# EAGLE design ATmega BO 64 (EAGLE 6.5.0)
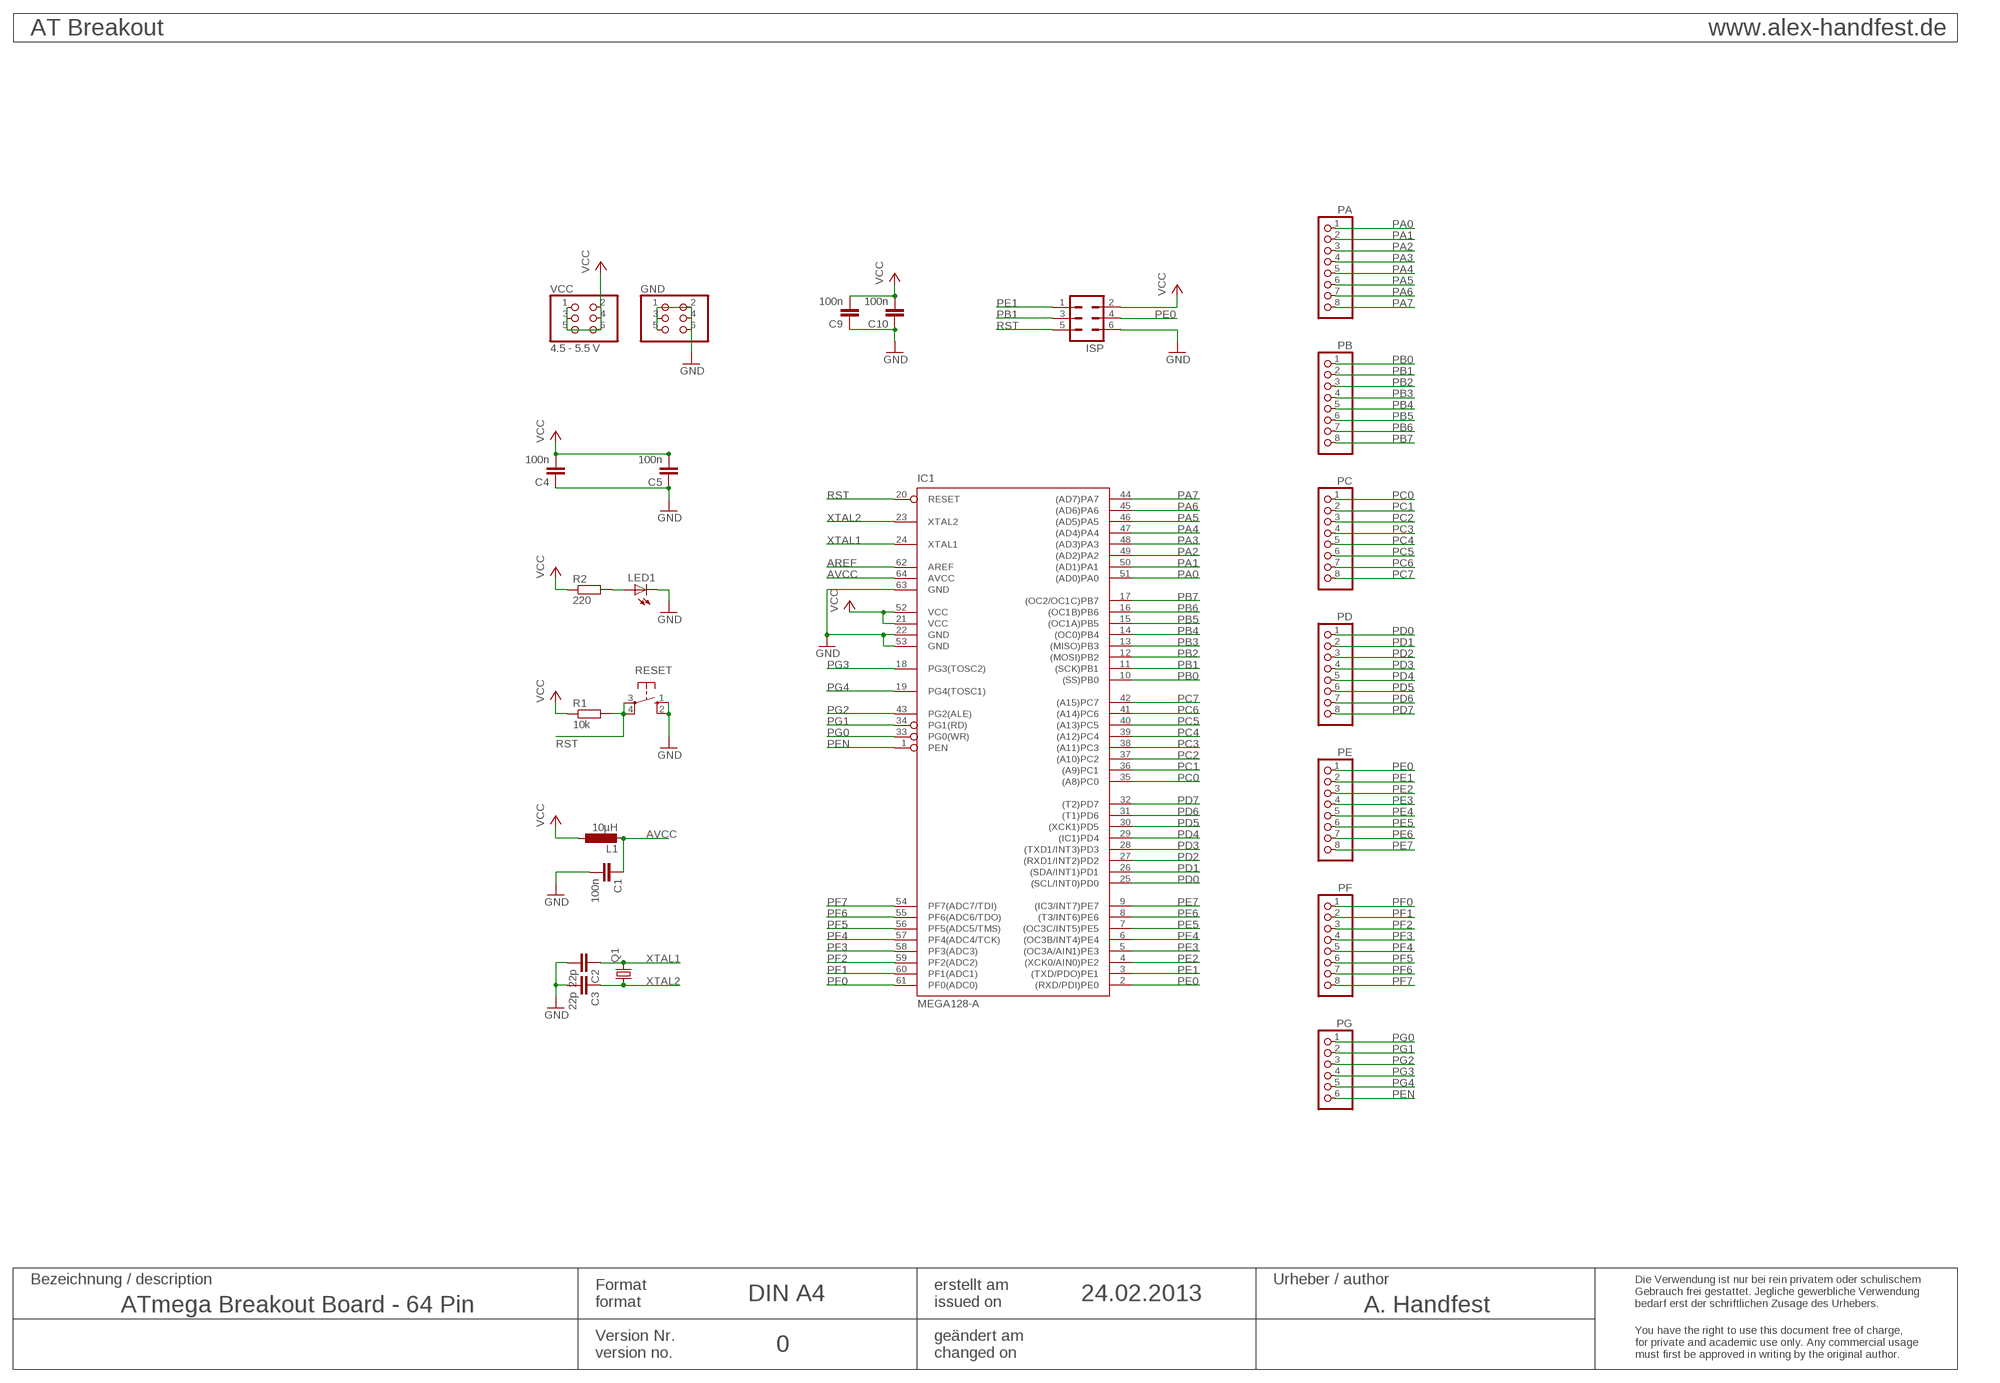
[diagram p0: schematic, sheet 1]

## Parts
C1  100n  C-EUC0805  [C0805]
C2  22p  C-EUC0805  [C0805]
C3  22p  C-EUC0805  [C0805]
C4  100n  C-EUC0805  [C0805]
C5  100n  C-EUC0805  [C0805]
C9  100n  C-EUC0805  [C0805]
C10  100n  C-EUC0805  [C0805]
GND  PINHD-2X3  [2X03]
IC1  MEGA128-A  [TQFP64]
ISP  ML6  [ML6]
L1  10µH  L-EUL2012C  [L2012C]
LED1  LEDCHIP-LED0805  [CHIP-LED0805]
PA  PINHD-1X8  [1X08]
PB  PINHD-1X8  [1X08]
PC  PINHD-1X8  [1X08]
PD  PINHD-1X8  [1X08]
PE  PINHD-1X8  [1X08]
PF  PINHD-1X8  [1X08]
PG  PINHD-1X6  [1X06]
Q1  CRYSTALCTS406  [CTS406]
R1  10k  R-EU_R0805  [R0805]
R2  220  R-EU_R0805  [R0805]
RESET  10-XX  [B3F-10XX]
VCC  4.5 - 5.5 V  PINHD-2X3  [2X03]

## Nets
AREF: IC1.62(AREF)
AVCC: C1.1 IC1.64(AVCC) L1.2
GND: C1.2 C2.2 C3.2 C4.1 C5.1 C9.1 C10.1 GND.1 GND.2 GND.3 GND.4 GND.5 GND.6 IC1.22(GND) IC1.53(GND) IC1.63(GND) ISP.6 LED1.C RESET.1(S) RESET.2(S1)
N$6: LED1.A R2.2
PA0: IC1.51((AD0)PA0) PA.1
PA1: IC1.50((AD1)PA1) PA.2
PA2: IC1.49((AD2)PA2) PA.3
PA3: IC1.48((AD3)PA3) PA.4
PA4: IC1.47((AD4)PA4) PA.5
PA5: IC1.46((AD5)PA5) PA.6
PA6: IC1.45((AD6)PA6) PA.7
PA7: IC1.44((AD7)PA7) PA.8
PB0: IC1.10((SS)PB0) PB.1
PB1: IC1.11((SCK)PB1) ISP.3 PB.2
PB2: IC1.12((MOSI)PB2) PB.3
PB3: IC1.13((MISO)PB3) PB.4
PB4: IC1.14((OC0)PB4) PB.5
PB5: IC1.15((OC1A)PB5) PB.6
PB6: IC1.16((OC1B)PB6) PB.7
PB7: IC1.17((OC2/OC1C)PB7) PB.8
PC0: IC1.35((A8)PC0) PC.1
PC1: IC1.36((A9)PC1) PC.2
PC2: IC1.37((A10)PC2) PC.3
PC3: IC1.38((A11)PC3) PC.4
PC4: IC1.39((A12)PC4) PC.5
PC5: IC1.40((A13)PC5) PC.6
PC6: IC1.41((A14)PC6) PC.7
PC7: IC1.42((A15)PC7) PC.8
PD0: IC1.25((SCL/INT0)PD0) PD.1
PD1: IC1.26((SDA/INT1)PD1) PD.2
PD2: IC1.27((RXD1/INT2)PD2) PD.3
PD3: IC1.28((TXD1/INT3)PD3) PD.4
PD4: IC1.29((IC1)PD4) PD.5
PD5: IC1.30((XCK1)PD5) PD.6
PD6: IC1.31((T1)PD6) PD.7
PD7: IC1.32((T2)PD7) PD.8
PE0: IC1.2((RXD/PDI)PE0) ISP.4 PE.1
PE1: IC1.3((TXD/PDO)PE1) ISP.1 PE.2
PE2: IC1.4((XCK0/AIN0)PE2) PE.3
PE3: IC1.5((OC3A/AIN1)PE3) PE.4
PE4: IC1.6((OC3B/INT4)PE4) PE.5
PE5: IC1.7((OC3C/INT5)PE5) PE.6
PE6: IC1.8((T3/INT6)PE6) PE.7
PE7: IC1.9((IC3/INT7)PE7) PE.8
PEN: IC1.1(PEN) PG.6
PF0: IC1.61(PF0(ADC0)) PF.1
PF1: IC1.60(PF1(ADC1)) PF.2
PF2: IC1.59(PF2(ADC2)) PF.3
PF3: IC1.58(PF3(ADC3)) PF.4
PF4: IC1.57(PF4(ADC4/TCK)) PF.5
PF5: IC1.56(PF5(ADC5/TMS)) PF.6
PF6: IC1.55(PF6(ADC6/TDO)) PF.7
PF7: IC1.54(PF7(ADC7/TDI)) PF.8
PG0: IC1.33(PG0(WR)) PG.1
PG1: IC1.34(PG1(RD)) PG.2
PG2: IC1.43(PG2(ALE)) PG.3
PG3: IC1.18(PG3(TOSC2)) PG.4
PG4: IC1.19(PG4(TOSC1)) PG.5
RST: IC1.20(RESET) ISP.5 R1.2 RESET.3(P) RESET.4(P1)
VCC: C4.2 C5.2 C9.2 C10.2 IC1.21(VCC) IC1.52(VCC) ISP.2 L1.1 R1.1 R2.1 VCC.1 VCC.2 VCC.3 VCC.4 VCC.5 VCC.6
XTAL1: C2.1 IC1.24(XTAL1) Q1.3
XTAL2: C3.1 IC1.23(XTAL2) Q1.1

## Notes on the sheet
- AT Breakout | www.alex-handfest.de
- Bezeichnung / description | Urheber / author
- Format | erstellt am
- DIN A4 | 24.02.2013
- format | issued on
- Die Verwendung ist nur bei rein privatem oder schulischem
  Gebrauch frei gestattet. Jegliche gewerbliche Verwendung 
  bedarf erst der schriftlichen Zusage des Urhebers.
- ATmega Breakout Board - 64 Pin | A. Handfest
- Version Nr. | geändert am
- 0
- version no. | changed on
- You have the right to use this document free of charge,
  for private and academic use only. Any commercial usage
  must first be approved in writing by the original author.

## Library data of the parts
C1-C5 C9 C10 = rcl:C-EU: CAPACITOR, European symbol
GND VCC = pinhead:PINHD-2X3: PIN HEADER
IC1 = atmel:MEGA128: MICROCONTROLLER 128 Kbytes FLASH 4 Kbytes SRAM 4 Kbytes EEPROM DUAL USART 8-channel 10 bit ADC Source: avr.lbr
ISP = con-harting-ml:ML6: HARTING
L1 = rcl:L-EU: INDUCTOR, European symbol
LED1 = led:LED: LED
PA PB PC PD PE PF = pinhead:PINHD-1X8: PIN HEADER
PG = pinhead:PINHD-1X6: PIN HEADER
Q1 = crystal:CRYSTAL: CRYSTAL; OC_FARNELL: unknown; OC_NEWARK: unknown
R1 R2 = rcl:R-EU_: RESISTOR, European symbol
RESET = switch-omron:10-XX: OMRON SWITCH

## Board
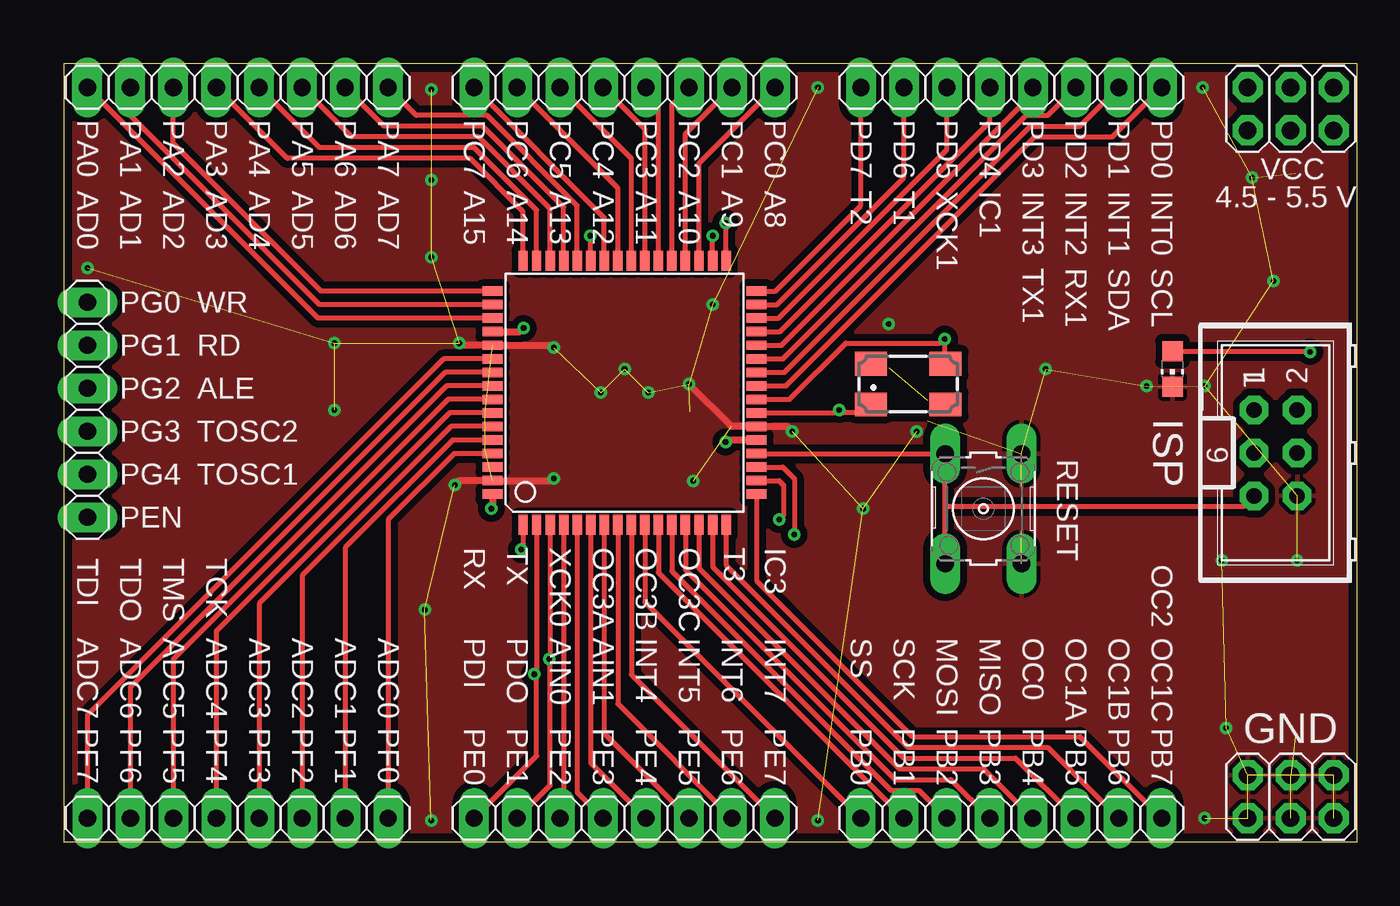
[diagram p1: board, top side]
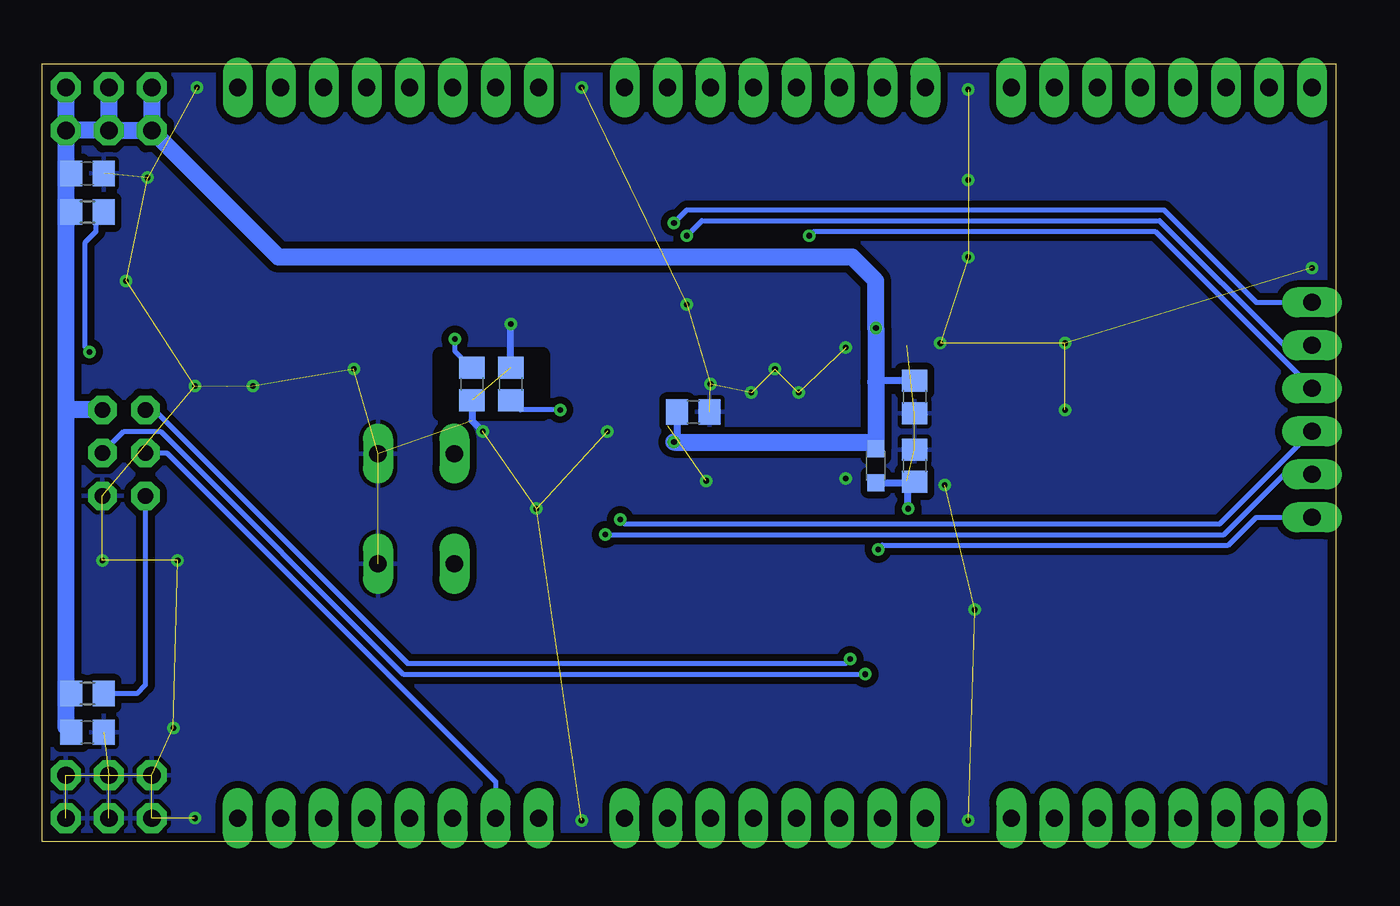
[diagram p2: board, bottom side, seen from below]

Size 76.45 x 45.97 mm. Coordinates in mm from the lower left corner, seen from the top.
Outline: 0,0 76.45,0 76.45,45.97 0,45.97 0,0
Copper layers (1*16): Top 0.035mm / dielectric 1.5mm / Bottom 0.035mm
Design rules "default *": minimum track width 10mil, minimum drill 24mil, track to track 8mil, track to pad 8mil, pad to pad 8mil, via to via 8mil, smd to smd 8mil, copper to edge 20mil, drill to drill 8mil, minimum pad ring 15mil, minimum via ring 8mil, stop-mask expansion 4mil, vias tented up to drill 20mil, thermal gap 10mil
tRestrict: area 46.9,25.3 to 53,28.8
bRestrict: area 46.9,25.3 to 53,28.8

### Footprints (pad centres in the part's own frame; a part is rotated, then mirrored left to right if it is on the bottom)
C0805 = smd 1.3 x 1.5: 1 -0.95,0; 2 0.95,0
2X03 = drill 1.016 octagon: 1 -2.54,-1.27; 2 -2.54,1.27; 3 0,-1.27; 4 0,1.27; 5 2.54,-1.27; 6 2.54,1.27
TQFP64 = smd 1.194 x 0.559: 1 -7.8,6; 2 -7.8,5.2; 3 -7.8,4.4; 4 -7.8,3.6; 5 -7.8,2.8; 6 -7.8,2; 7 -7.8,1.2; 8 -7.8,0.4; 9 -7.8,-0.4; 10 -7.8,-1.2; 11 -7.8,-2; 12 -7.8,-2.8; 13 -7.8,-3.6; 14 -7.8,-4.4; 15 -7.8,-5.2; 16 -7.8,-6; 33 7.8,-6; 34 7.8,-5.2; 35 7.8,-4.4; 36 7.8,-3.6; 37 7.8,-2.8; 38 7.8,-2; 39 7.8,-1.2; 40 7.8,-0.4; 41 7.8,0.4; 42 7.8,1.2; 43 7.8,2; 44 7.8,2.8; 45 7.8,3.6; 46 7.8,4.4; 47 7.8,5.2; 48 7.8,6 | smd 0.559 x 1.194: 17 -6,-7.8; 18 -5.2,-7.8; 19 -4.4,-7.8; 20 -3.6,-7.8; 21 -2.8,-7.8; 22 -2,-7.8; 23 -1.2,-7.8; 24 -0.4,-7.8; 25 0.4,-7.8; 26 1.2,-7.8; 27 2,-7.8; 28 2.8,-7.8; 29 3.6,-7.8; 30 4.4,-7.8; 31 5.2,-7.8; 32 6,-7.8; 49 6,7.8; 50 5.2,7.8; 51 4.4,7.8; 52 3.6,7.8; 53 2.8,7.8; 54 2,7.8; 55 1.2,7.8; 56 0.4,7.8; 57 -0.4,7.8; 58 -1.2,7.8; 59 -2,7.8; 60 -2.8,7.8; 61 -3.6,7.8; 62 -4.4,7.8; 63 -5.2,7.8; 64 -6,7.8
ML6 = drill 0.914 octagon: 1 -2.54,-1.27; 2 -2.54,1.27; 3 0,-1.27; 4 0,1.27; 5 2.54,-1.27; 6 2.54,1.27
L2012C = smd 1 x 1: 1 -1,0; 2 1,0
CHIP-LED0805 = smd 1.2 x 1.2: A 0,-1.05; C 0,1.05
1X08 = drill 1.016 long: 1 -8.89,0; 2 -6.35,0; 3 -3.81,0; 4 -1.27,0; 5 1.27,0; 6 3.81,0; 7 6.35,0; 8 8.89,0
1X06 = drill 1.016 long: 1 -6.35,0; 2 -3.81,0; 3 -1.27,0; 4 1.27,0; 5 3.81,0; 6 6.35,0
CTS406 = smd 1.9 x 1.4: 1 -2.2,-1.2; 2 2.2,-1.2; 3 2.2,1.2; 4 -2.2,1.2
R0805 = smd 1.3 x 1.5: 1 -0.95,0; 2 0.95,0
B3F-10XX = drill 1.016 long: 1 -3.251,2.261; 2 3.251,2.261; 3 -3.251,-2.261; 4 3.251,-2.261

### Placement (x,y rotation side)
C1  24.89,22.23 90 bottom
C2  51.05,27.05 270 bottom
C3  48.77,27.05 90 bottom
C4  37.97,25.4 180 bottom
C5  24.89,26.29 90 bottom
C9  73.79,6.48 180 bottom
C10  73.79,39.5 180 bottom
GND  72.52,2.67 0 top
IC1  33.15,26.54 90 top
ISP  71.63,22.99 270 top
L1  27.18,22.23 270 bottom
LED1  65.53,27.94 180 top
PA  10.29,44.58 0 top
PB  56.01,1.4 0 top
PC  33.15,44.58 180 top
PD  56.01,44.58 180 top
PE  33.15,1.4 0 top
PF  10.29,1.4 180 top
PG  1.4,25.53 270 top
Q1  49.91,27.05 0 top
R1  73.79,8.76 0 bottom
R2  73.79,37.21 0 bottom
RESET  54.36,19.68 270 top
VCC  72.52,43.31 0 top

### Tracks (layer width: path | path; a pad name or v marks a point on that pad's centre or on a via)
AVCC  (via drill 0.33)
  Top 0.406: IC1.64 25.35,19.76 v25.27,19.68
  Bottom 0.406: L1.2 25.4,21.23 | 25.4,21.23 24.94,21.23 C1.1 | v25.27,19.68 25.27,21.1 25.4,21.23
GND  (via drill 0.33)  (45 unrouted)
  Top 0.406: v23.37,29.46 23.49,29.34 IC1.53 28.82,29.34 v28.96,29.21 | v23.11,21.08 23.38,21.34 IC1.63 28.84,21.34 v28.96,21.46 | v36.96,27.05 39.47,24.54 IC1.22 42.77,24.54 v43.05,24.26
  Bottom 0.406: C2.2 51.05,24.89 v50.42,24.26 | C3.2 v48.77,30.61
  other vias: 31.75,26.54 33.15,27.94 34.54,26.54 37.21,21.34 38.35,31.75 70.23,39.24 67.44,26.92 64.01,26.92 72.9,16.64 68.45,16.64 68.71,6.73 44.58,1.27 67.44,1.4 21.72,1.27 1.4,33.91 21.72,44.45 21.72,39.12 21.72,34.54 16,29.46 16,25.53 44.58,44.58 67.31,44.58 58.04,27.94 47.24,19.68 21.34,13.72 71.5,33.15
  pour Bottom (isolate 0.406): -0.25,46.23 76.71,46.23 76.71,-0.25 -0.25,-0.25
  pour Top (isolate 0.406): -0.25,46.23 76.71,46.23 76.71,-0.25 -0.25,-0.25
N$6  (via drill 0.33)
  Top 0.305: LED1.A 73.63,28.99 v73.66,28.96
  Bottom 0.305: v73.66,28.96 73.91,29.21 73.91,35.43 73.28,36.07 73.28,36.77 R2.2
PA0
  Top 0.305: IC1.51 15.03,30.94 PA.1
PA1
  Top 0.305: IC1.50 15.12,31.74 3.94,42.93 PA.2
PA2
  Top 0.305: IC1.49 15.21,32.54 6.48,41.27 PA.3
PA3
  Top 0.305: IC1.48 27.15,37.24 24,40.39 13.21,40.39 PA.4
PA4
  Top 0.305: IC1.47 27.95,37.33 24.26,41.02 15.11,41.02 PA.5
PA5
  Top 0.305: IC1.46 28.75,37.42 24.51,41.66 17.02,41.66 PA.6
PA6
  Top 0.305: IC1.45 29.55,37.51 24.77,42.29 18.92,42.29 PA.7
PA7
  Top 0.305: IC1.44 30.35,37.6 25.02,42.93 20.83,42.93 PA.8
PB0
  Top 0.305: IC1.10 34.35,14.17 PB.1
PB1
  Top 0.305: IC1.11 35.15,15.91 PB.2
  Bottom 0.305: ISP.3 69.09,22.99 49.66,3.56 PB.2
PB2
  Top 0.305: IC1.12 35.95,16 48.9,3.05 50.55,3.05 PB.3
PB3
  Top 0.305: IC1.13 36.75,16.09 49.15,3.68 52.45,3.68 PB.4
PB4
  Top 0.305: IC1.14 37.55,16.17 49.4,4.32 54.36,4.32 PB.5
PB5
  Top 0.305: IC1.15 38.35,16.26 49.66,4.95 56.26,4.95 PB.6
PB6
  Top 0.305: IC1.16 39.15,16.35 49.91,5.59 58.17,5.59 PB.7
PB7
  Top 0.305: IC1.17 40.95,15.44 50.16,6.22 60.07,6.22 PB.8
PC0
  Top 0.305: IC1.35 37.55,40.09 PC.1
PC1
  Top 0.305: IC1.36 36.75,41.83 PC.2
PC2
  Top 0.305: IC1.37 35.95,43.57 PC.3
PC3
  Top 0.305: IC1.38 35.15,43.85 PC.4
PC4
  Top 0.305: IC1.39 34.35,42.11 PC.5
PC5
  Top 0.305: IC1.40 33.55,40.37 PC.6
PC6
  Top 0.305: IC1.41 32.75,38.63 PC.7
PC7
  Top 0.305: IC1.42 31.95,36.89 PC.8
PD0
  Top 0.305: IC1.25 42.69,26.94 57.4,41.66 61.98,41.66 PD.1
PD1
  Top 0.305: IC1.26 42.6,27.74 57.15,42.29 60.07,42.29 PD.2
PD2
  Top 0.305: IC1.27 42.51,28.54 56.9,42.93 58.17,42.93 PD.3
PD3
  Top 0.305: IC1.28 42.42,29.34 57.28,44.2 PD.4
PD4
  Top 0.305: IC1.29 42.34,30.14 54.74,42.55 PD.5
PD5
  Top 0.305: IC1.30 42.25,30.94 52.2,40.89 PD.6
PD6
  Top 0.305: IC1.31 42.16,31.74 49.66,39.24 PD.7
PD7
  Top 0.305: IC1.32 42.07,32.54 47.12,37.59 PD.8
PE0  (via drill 0.33)
  Top 0.305: PE.1 27.95,5.09 27.95,9.77 v27.81,9.91 27.95,10.04 IC1.2
  Bottom 0.305: ISP.4 71.63,24.26 69.47,24.26 55.12,9.91 v27.81,9.91
PE1  (via drill 0.33)
  Top 0.305: PE.2 28.75,3.35 28.75,10.75 v28.7,10.79 28.75,10.84 IC1.3
  Bottom 0.305: ISP.1 69.85,25.53 54.86,10.54 28.96,10.54 v28.7,10.79
PE2
  Top 0.305: IC1.4 29.55,1.61 PE.3
PE3
  Top 0.305: IC1.5 30.35,2.93 PE.4
PE4
  Top 0.305: IC1.6 31.15,4.67 PE.5
PE5
  Top 0.305: IC1.7 31.95,6.41 PE.6
PE6
  Top 0.305: IC1.8 32.75,8.15 PE.7
PE7
  Top 0.305: IC1.9 33.55,9.89 PE.8
PEN  (via drill 0.33)
  Top 0.305: IC1.1 27.15,17.37 v27.05,17.27
  Bottom 0.305: v27.05,17.27 26.8,17.53 6.35,17.53 4.7,19.18 PG.6
PF0
  Top 0.305: IC1.61 23.07,22.94 19.18,19.05 PF.1
PF1
  Top 0.305: IC1.60 22.98,23.74 16.64,17.4 PF.2
PF2
  Top 0.305: IC1.59 22.89,24.54 14.1,15.75 PF.3
PF3
  Top 0.305: IC1.58 22.8,25.34 11.56,14.1 PF.4
PF4
  Top 0.305: IC1.57 22.71,26.14 9.02,12.45 PF.5
PF5
  Top 0.305: IC1.56 22.62,26.94 6.48,10.79 PF.6
PF6
  Top 0.305: IC1.55 22.54,27.74 3.94,9.14 PF.7
PF7
  Top 0.305: IC1.54 22.45,28.54 1.4,7.49 PF.8
PG0  (via drill 0.33)
  Top 0.305: IC1.33 39.15,36.55 v39.12,36.58
  Bottom 0.305: v39.12,36.58 38.35,37.34 10.16,37.34 4.7,31.88 PG.1
PG1  (via drill 0.33)
  Top 0.305: IC1.34 v38.35,35.81
  Bottom 0.305: v38.35,35.81 37.47,36.7 10.41,36.7 3.05,29.34 PG.2
PG2  (via drill 0.33)
  Top 0.305: IC1.43 31.15,35.78 v31.11,35.81
  Bottom 0.305: v31.11,35.81 30.86,36.07 10.67,36.07 PG.3
PG3  (via drill 0.33)
  Top 0.305: IC1.18 42.28,21.34 42.55,21.08 42.55,19.3 v42.29,19.05
  Bottom 0.305: v42.29,19.05 42.04,18.8 6.86,18.8 PG.4
PG4  (via drill 0.33)
  Top 0.305: IC1.19 42.5,22.14 43.18,21.46 v43.18,18.16
  Bottom 0.305: v43.18,18.16 6.6,18.16 3.05,21.72 PG.5
RST
  Top 0.305: IC1.20 52.09,22.94 RESET.3 52.09,19.81 | RESET.4 52.09,19.81 | ISP.5 69.72,19.81 52.09,19.81
  Bottom 0.305: ISP.5 70.36,9.27 70.87,8.76 R1.2
VCC  (via drill 0.33)
  Top 0.406: IC1.52 26.97,30.14 v27.18,30.35 | IC1.21 39.24,23.74 v39.12,23.62
  Bottom 0.406: C10.2 75.06,39.5 | R2.1 74.93,37.21 75.06,37.08 | R1.1 74.93,8.76 75.06,8.64 | C5.2 27.12,27.24 27.18,27.18 | C4.2 38.92,23.82 v39.12,23.62
  Bottom 1.016: VCC.5 75.06,39.5 75.06,37.08 75.06,25.4 | 75.06,25.4 75.06,8.64 75.06,6.8 C9.2 | ISP.2 74.93,25.53 75.06,25.4 | VCC.1 62.48,34.54 28.57,34.54 27.18,33.15 v27.18,30.35 27.18,27.18 27.18,23.75 | VCC.3 VCC.1 | VCC.3 VCC.5 | VCC.2 VCC.1 | VCC.4 VCC.3 | VCC.6 VCC.5 | v39.12,23.62 27.3,23.62 27.18,23.75 | 27.18,23.75 L1.1
XTAL1  (via drill 0.33)
  Top 0.305: IC1.24 42.91,26.14 46.23,29.46 51.82,29.46 v52.07,29.72 52.07,28.29 Q1.3
  Bottom 0.305: v52.07,29.72 52.07,29.02 C2.1
XTAL2  (via drill 0.33)
  Top 0.305: IC1.23 45.66,25.34 | 45.66,25.34 v45.85,25.53 | Q1.1 47.2,25.34 45.66,25.34
  Bottom 0.305: v45.85,25.53 48.19,25.53 C3.1

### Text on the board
tNames: PA0 | PA1 | PA2 | PA3 | PA4 | PA5 | PA6 | PA7 | PC7 | PC6 | PC5 | PC4 | PC3 | PC2 | PC1 | PC0 | PD7 | PD6 | PD5 | PD4 | PD3 | PD2 | PD1 | PD0 | AD0 | AD1 | AD2 | AD3 | AD4 | AD5 | AD6 | AD7 | A15 | A14 | A13 | A12 | A11 | A10 | A9 | A8 | T2 | T1 | XCK1 | IC1 | INT3 | INT2 | INT1 | INT0 | TX1 | RX1 | SDA | SCL | PG0 | WR | PG1 | RD | 1 | PG2 | ALE | PG3 | TOSC2 | PG4 | TOSC1 | PEN | TDI | TDO | TMS | TCK | RX | TX | XCK0 | OC3A | OC3B | OC3C | T3 | IC3 | OC2 | ADC7 | ADC6 | ADC5 | ADC4 | ADC3 | ADC2 | ADC1 | ADC0 | PDI | PDO | AIN0 | AIN1 | INT4 | INT5 | INT6 | INT7 | SS | SCK | MOSI | MISO | OC0 | OC1A | OC1B | OC1C | PF7 | PF6 | PF5 | PF4 | PF3 | PF2 | PF1 | PF0 | PE0 | PE1 | PE2 | PE3 | PE4 | PE5 | PE6 | PE7 | PB0 | PB1 | PB2 | PB3 | PB4 | PB5 | PB6 | PB7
